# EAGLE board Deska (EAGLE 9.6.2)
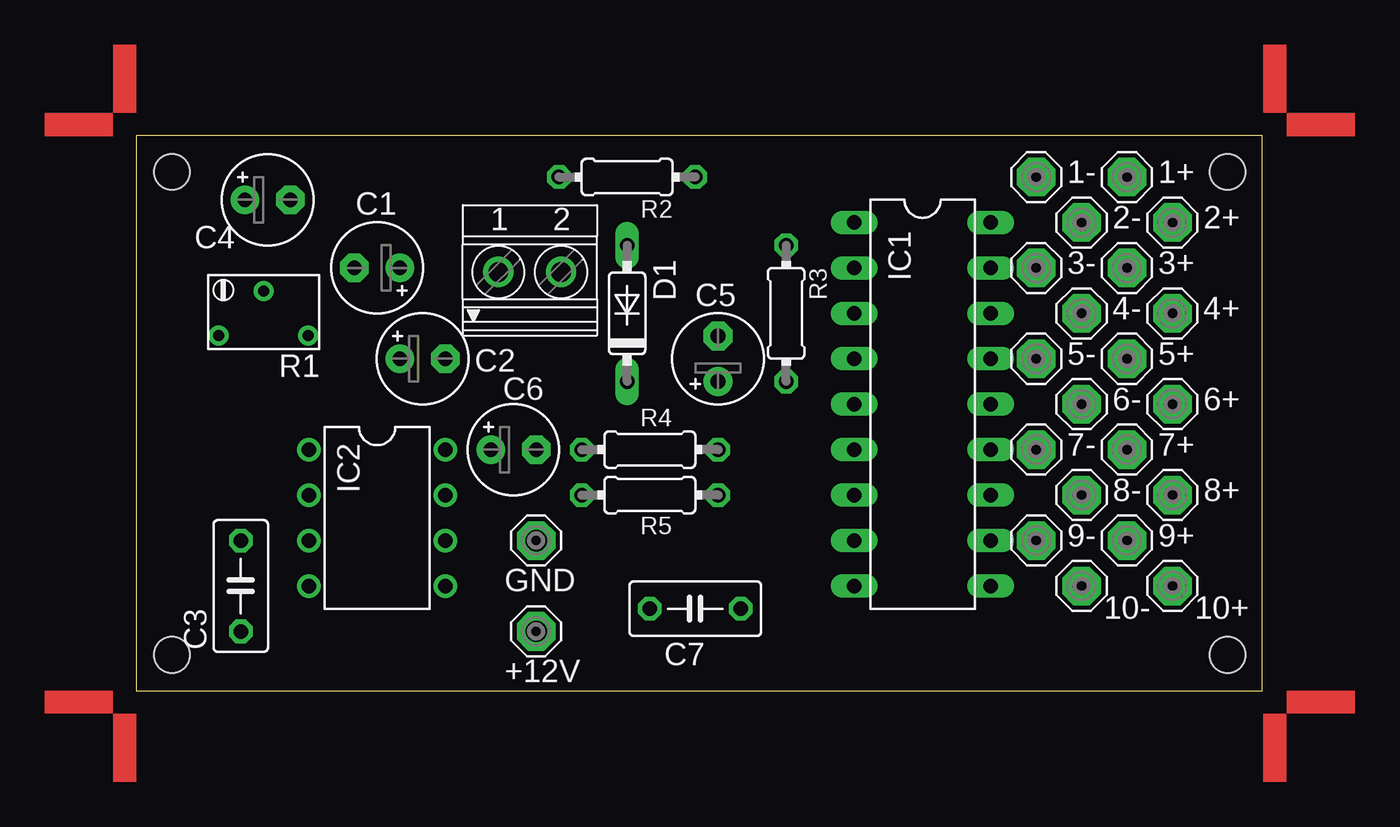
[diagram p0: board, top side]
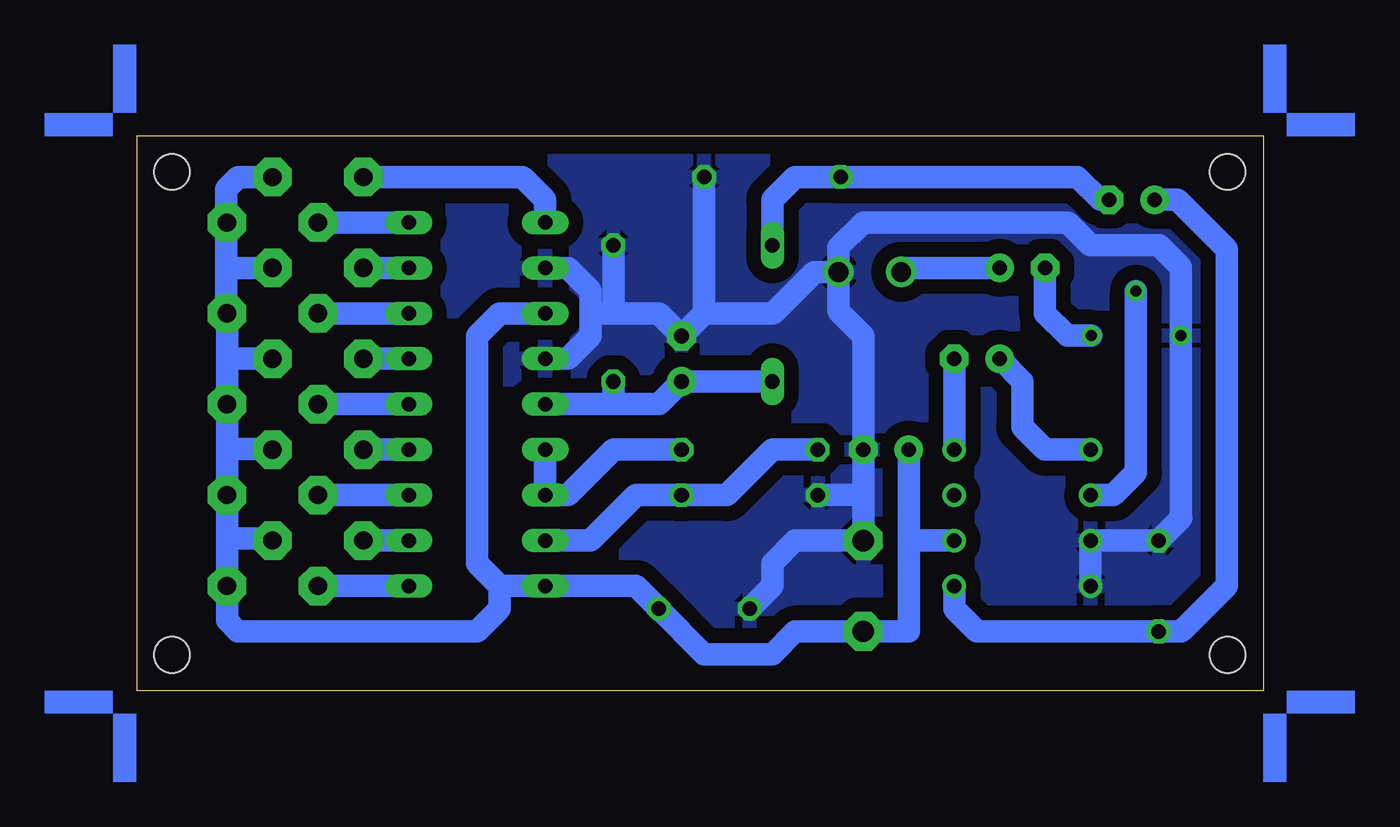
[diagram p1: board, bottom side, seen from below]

Size 62.94 x 31.01 mm. Coordinates in mm from the lower left corner, seen from the top.
Outline: 0,0 62.94,0 62.94,31.01 0,31.01 0,0
Copper layers (1*16): Top 0.035mm / dielectric 1.5mm / Bottom 0.035mm
Design rules "default": minimum track width 6mil, minimum drill 0.35mm, track to track 6mil, track to pad 6mil, pad to pad 6mil, via to via 6mil, smd to smd 6mil, copper to edge 40mil, drill to drill 6mil, minimum pad ring 10mil, minimum via ring 8mil, stop-mask expansion 4mil, vias tented up to drill 0mil, thermal gap 10mil
Holes 2 mm at 2,29 61,2 61,29 2,2

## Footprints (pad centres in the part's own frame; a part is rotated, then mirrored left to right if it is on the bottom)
MCS10B = drill 1.016 pad 2.159 octagon: MP 0,0
MCS08 = drill 1.194 pad 2.159 octagon: MP 0,0
E2,5-5 = drill 0.813 pad 1.6: + -1.27,0 | drill 0.813 pad 1.6 octagon: - 1.27,0
C050-030X075 = drill 0.813 octagon: 1 -2.54,0; 2 2.54,0
DO35-7 = drill 0.813 long: A 3.81,0; C -3.81,0
DIL18 = drill 0.813 long: 1 -10.16,-3.81; 2 -7.62,-3.81; 3 -5.08,-3.81; 4 -2.54,-3.81; 5 0,-3.81; 6 2.54,-3.81; 7 5.08,-3.81; 8 7.62,-3.81; 9 10.16,-3.81; 10 10.16,3.81; 11 7.62,3.81; 12 5.08,3.81; 13 2.54,3.81; 14 0,3.81; 15 -2.54,3.81; 16 -5.08,3.81; 17 -7.62,3.81; 18 -10.16,3.81
DIL08 = drill 0.813 pad 1.27: 1 -3.81,-3.81; 2 -1.27,-3.81; 3 1.27,-3.81; 4 3.81,-3.81; 5 3.81,3.81; 6 1.27,3.81; 7 -1.27,3.81; 8 -3.81,3.81
RTRIM74W = drill 0.61: 1 -1.25,-2.5; 2 1.25,0; 3 -1.25,2.5
0204/7 = drill 0.813 octagon: 1 -3.81,0; 2 3.81,0
1751248 = drill 1.1 pad 1.7: 1 -1.75,-0.1; 2 1.75,-0.1

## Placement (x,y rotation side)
1+  MCS10B  [MCS10B]  55.38,28.71 0 top
1-  MCS10B  [MCS10B]  50.3,28.71 0 top
2+  MCS10B  [MCS10B]  57.92,26.17 0 top
2-  MCS10B  [MCS10B]  52.84,26.17 0 top
3+  MCS10B  [MCS10B]  55.38,23.63 0 top
3-  MCS10B  [MCS10B]  50.3,23.63 0 top
4+  MCS10B  [MCS10B]  57.92,21.09 0 top
4-  MCS10B  [MCS10B]  52.84,21.09 0 top
5+  MCS10B  [MCS10B]  55.38,18.55 0 top
5-  MCS10B  [MCS10B]  50.3,18.55 0 top
6+  MCS10B  [MCS10B]  57.92,16.01 0 top
6-  MCS10B  [MCS10B]  52.84,16.01 0 top
7+  MCS10B  [MCS10B]  55.38,13.47 0 top
7-  MCS10B  [MCS10B]  50.3,13.47 0 top
8+  MCS10B  [MCS10B]  57.92,10.93 0 top
8-  MCS10B  [MCS10B]  52.84,10.93 0 top
9+  MCS10B  [MCS10B]  55.38,8.39 0 top
9-  MCS10B  [MCS10B]  50.3,8.39 0 top
10+  MCS10B  [MCS10B]  57.92,5.85 0 top
10-  MCS10B  [MCS10B]  52.84,5.85 0 top
+12V  MCS08  [MCS08]  22.36,3.31 0 top
C1  [E2,5-5]  13.47,23.63 180 top
C2  [E2,5-5]  16.01,18.55 0 top
C3  [C050-030X075]  5.85,5.85 90 top
C4  [E2,5-5]  7.35,27.44 0 top
C5  [E2,5-5]  32.52,18.55 90 top
C6  [E2,5-5]  21.09,13.47 0 top
C7  [C050-030X075]  31.25,4.58 180 top
D1  [DO35-7]  27.44,21.09 90 top
GND  MCS08  [MCS08]  22.36,8.39 0 top
IC1  LM3915  [DIL18]  43.95,16.01 270 top
IC2  LM386N-1  [DIL08]  13.47,9.66 270 top
R1  [RTRIM74W]  7.12,21.09 90 top
R2  [0204/7]  27.44,28.71 180 top
R3  [0204/7]  36.33,21.09 270 top
R4  [0204/7]  28.71,13.47 0 top
R5  [0204/7]  28.71,10.93 0 top
U$1  [ANGLE-SW1-16]  63,31 0 top
U$2  [ANGLE-SW1-16]  0,31 90 top
U$3  [ANGLE-SW1-16]  0,0 180 top
U$4  [ANGLE-SW1-16]  63,0 270 top
X1  1751248  [1751248]  22,23.5 0 top

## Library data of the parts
1+ 1- 2+ 2- 3+ 3- 4+ 4- 5+ 5- 6+ 6- 7+ 7- 8+ 8- 9+ 9- 10+ 10- +12V GND = solpad
C1-C7 = rcl; SPICEPREFIX: C
D1 = diode
IC1 = national-semiconductor
IC2 = linear
R1 = rcl; SPICEMODEL: X; SPICEPREFIXL: POT
R2-R5 = rcl; SPICEPREFIX: R
U$1-U$4 = marks
X1 = con-phoenix-350; OC_FARNELL: unknown; OC_NEWARK: unknown

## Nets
GND: C3.2 C5.- C6.- C7.2 GND.MP IC1.2 IC1.4 IC2.3 IC2.4 R1.3 R2.1 R3.1 R5.1 X1.2
N$1: C2.+ IC2.1
N$2: C2.- IC2.8
N$3: C3.1 C4.+ IC2.5
N$4: C4.- D1.A R2.2
N$5: C5.+ D1.C IC1.5 R3.2
N$6: IC2.2 R1.2
N$7: C1.- R1.1
N$8: C1.+ X1.1
N$10: IC1.8 R4.1 R5.2
N$11: IC1.6 IC1.7 R4.2
N$12: 1+.MP 2+.MP 3+.MP 4+.MP 5+.MP 6+.MP 7+.MP 8+.MP 9+.MP 10+.MP +12V.MP C6.+ C7.1 IC1.3 IC1.9 IC2.6
N$13: 1-.MP IC1.1
N$14: 2-.MP IC1.18
N$15: 3-.MP IC1.17
N$16: 4-.MP IC1.16
N$17: 5-.MP IC1.15
N$18: 6-.MP IC1.14
N$19: 7-.MP IC1.13
N$20: 8-.MP IC1.12
N$21: 9-.MP IC1.11
N$22: 10-.MP IC1.10

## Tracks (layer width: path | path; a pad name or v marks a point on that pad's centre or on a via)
GND
  Bottom 1.27: IC2.4 IC2.3 C3.2 4.58,9.66 4.62,9.7 R1.3 4.62,23.67 5.85,24.9 9.66,24.9 10.93,26.17 22.36,26.17 23.75,24.78 X1.2 | 22.36,10.93 C6.- 22.36,19.82 23.75,21.21 X1.2 | 22.36,10.93 GND.MP 26.17,8.39 27.44,7.12 27.44,5.85 C7.2 | IC1.4 38.87,18.55 37.6,19.82 37.6,21.09 | 37.6,21.09 37.6,22.36 38.87,23.63 IC1.2 | R2.1 31.25,21.09 | 31.25,21.09 C5.- 33.79,21.09 36.33,21.09 | 36.33,21.09 37.6,21.09 | R3.1 36.33,21.09 | R5.1 22.36,10.93 | X1.2 25.1,23.4 27.41,21.09 31.25,21.09
  pour Bottom (isolate 0.813): 0,0 63,0 63,31 0,31
N$1
  Bottom 1.27: C2.+ 13.47,17.28 13.47,14.74 12.2,13.47 IC2.1
N$2
  Bottom 1.27: C2.- IC2.8
N$3
  Bottom 1.27: IC2.5 17.28,4.58 16.01,3.31 C3.1 4.58,3.31 2.04,5.85 2.04,24.67 4.81,27.44 C4.+
N$4
  Bottom 1.27: C4.- 9.12,27.44 10.39,28.71 R2.2 26.17,28.71 27.44,27.44 D1.A
N$5
  Bottom 1.27: D1.C C5.+ 33.79,16.01 36.33,16.01 | IC1.5 36.33,16.01 | R3.2 36.33,16.01
N$6
  Bottom 1.27: IC2.2 8.39,10.93 7.12,12.2 R1.2
N$7
  Bottom 1.27: R1.1 10.95,19.84 12.2,21.09 C1.-
N$8
  Bottom 1.27: C1.+ 20.02,23.63 X1.1
N$10
  Bottom 1.27: IC1.8 37.6,8.39 35.06,10.93 R5.2 29.98,10.93 27.44,13.47 R4.1
N$11
  Bottom 1.27: IC1.6 IC1.7 38.87,10.93 36.33,13.47 R4.2
N$12
  Bottom 1.27: IC2.6 19.82,8.39 | 19.82,8.39 C6.+ | 19.82,8.39 19.82,3.31 +12V.MP 26.17,3.31 27.44,2.04 31.25,2.04 C7.1 35.06,5.85 IC1.9 42.68,5.85 | 42.68,5.85 43.95,7.12 43.95,19.82 42.68,21.09 IC1.3 | 57.96,26.17 57.96,23.63 | 57.96,23.63 57.96,21.09 4+.MP 57.92,18.5 | 42.68,5.85 42.68,4.58 43.95,3.31 57.31,3.31 57.92,3.92 10+.MP 57.92,8.5 | 2+.MP 57.96,26.17 | 3+.MP 57.96,23.63 | 1+.MP 57.29,28.71 57.96,28.04 57.96,26.17 | 57.92,18.5 6+.MP 57.92,13.5 | 57.92,13.5 8+.MP 57.92,8.5 | 9+.MP 55.49,8.5 57.92,8.5 | 7+.MP 55.41,13.5 57.92,13.5 | 5+.MP 57.87,18.55 57.92,18.5
N$13
  Bottom 1.27: IC1.1 40.14,27.44 41.41,28.71 1-.MP
N$14
  Bottom 1.27: IC1.18 2-.MP
N$15
  Bottom 1.27: IC1.17 3-.MP
N$16
  Bottom 1.27: IC1.16 4-.MP
N$17
  Bottom 1.27: IC1.15 5-.MP
N$18
  Bottom 1.27: IC1.14 6-.MP
N$19
  Bottom 1.27: IC1.13 7-.MP
N$20
  Bottom 1.27: IC1.12 8-.MP
N$21
  Bottom 1.27: IC1.11 9-.MP
N$22
  Bottom 1.27: IC1.10 10-.MP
